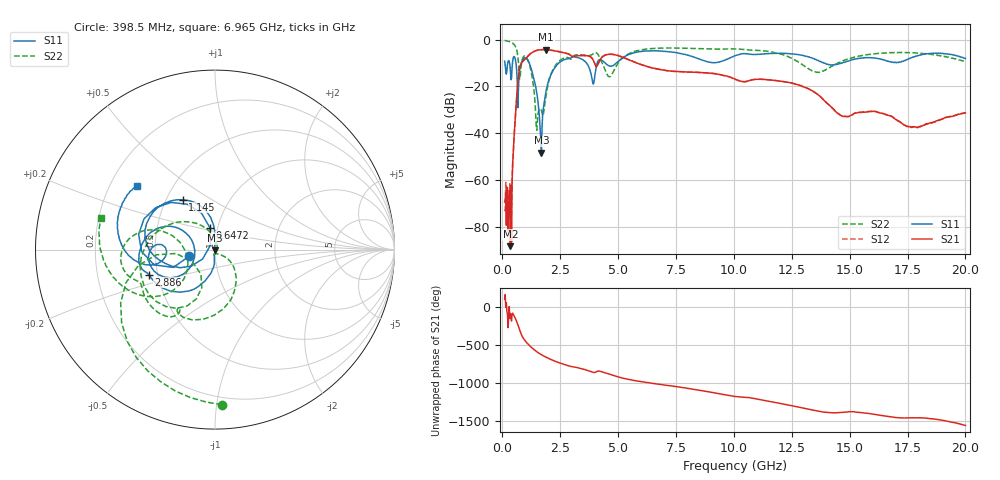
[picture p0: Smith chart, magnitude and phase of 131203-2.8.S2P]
!  2-Port S-parameters saved by WinCal
! VAR MeasName=S-Parameters (CALIBRATED_DATA) read from VNA (N5244A)
! VAR MeasDate=4/4/2013 3:56:53 PM
! VAR NAME=131203-2.8
! VAR FILENAME=131203-2.8.S2P
! VAR DATE=4/4/2013 3:56:53 PM
! VAR PHYS_PORTS=1,2
# Hz S MA R 50
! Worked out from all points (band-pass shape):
!   801 points, 100 MHz to 20 GHz, reference 50 ohm
!   highest |S21| = -4.27 dB at 1.891 GHz (marker M1); lowest = -88.1 dB at 348.8 MHz (marker M2)
!   |S21| within 3 dB of the highest: 1.086 GHz to 3.794 GHz (2.708 GHz wide, 111 % of centre); 4.335 GHz to 5.126 GHz (791.1 MHz wide, 16.7 % of centre)
!   lowest |S11| = -48.3 dB at 1.692 GHz (marker M3), VSWR 1.01, Z = 49.8 - j0.317 ohm
!   |S11| at or under -10 dB: 1.162 GHz to 2.442 GHz (1.279 GHz wide, 71 % of centre); 4.444 GHz to 4.926 GHz (482.2 MHz wide, 10.3 % of centre); 13.88 GHz to 14.65 GHz (768.2 MHz wide, 5.38 % of centre)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
!   |S22| runs from -38.7 to -0.4 dB; largest |S21 - S12| = 0.0032
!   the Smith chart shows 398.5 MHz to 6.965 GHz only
!   S11 on the Smith chart (normalised r, x): 398.5 MHz: 0.75, -0.06; 647.2 MHz: 0.92, +0.22; 1.145 GHz: 0.61, +0.38; 2.886 GHz: 0.44, -0.15; 6.965 GHz: 0.31, +0.32
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1e8  0.3458 152.9  0.0003482 99.3  0.0002348 153.8  0.9574 -22.2
3.4875e8  0.2226 142.1  3.945e-05 -90.0  0.0002087 -95.9  0.8884 -76.1
3.985e8  0.148 -165.5  4.834e-05 171.4  0.0001809 -136.6  0.8644 -87.5
6.4725e8  0.1224 102.9  0.08681 144.1  0.08681 144.2  0.5297 -159.6
8.71125e8  0.3637 -179.1  0.3392 -35.7  0.3397 -35.7  0.3914 -123.3
1.14475e9  0.3314 123.0  0.4632 -142.4  0.4645 -142.3  0.3222 158.9
1.468125e9  0.08422 87.8  0.5835 133.2  0.585 133.3  0.01395 23.8
1.692e9  0.003863 -124.5  0.6073 88.6  0.6087 88.6  0.03066 -106.3
1.891e9  0.08059 -92.5  0.6116 55.7  0.6132 55.7  0.06436 -36.6
2.264125e9  0.2508 -118.2  0.5789 5.0  0.5803 4.9  0.2646 -67.0
2.886e9  0.3953 -159.4  0.4869 -59.2  0.4885 -59.3  0.4017 -121.7
3.43325e9  0.3827 168.0  0.4562 -96.1  0.4574 -96.2  0.4706 -145.5
3.905875e9  0.1208 168.0  0.3813 -140.8  0.382 -140.9  0.4901 -160.9
4.62725e9  0.2742 179.2  0.4856 -168.8  0.4874 -169.1  0.1613 -166.6
5.3735e9  0.458 -173.1  0.3877 129.2  0.3884 129.0  0.472 -146.8
6.741625e9  0.5739 146.1  0.2327 61.3  0.2329 61.1  0.6551 169.8
6.9655e9  0.5632 140.8  0.2228 51.9  0.2225 51.7  0.6596 164.6
1.005e10  0.452 130.5  0.1438 -99.8  0.1439 -100.3  0.6318 113.2
1.338325e10  0.4023 74.3  0.08105 83.2  0.08107 83.3  0.2148 77.6
1.467675e10  0.3159 92.5  0.02348 51.2  0.02348 50.6  0.3442 113.6
1.669162e10  0.3416 72.6  0.024 -2.9  0.02395 -3.3  0.5187 85.9
2e10  0.3951 34.4  0.0274 -120.7  0.02731 -120.6  0.3418 51.3
